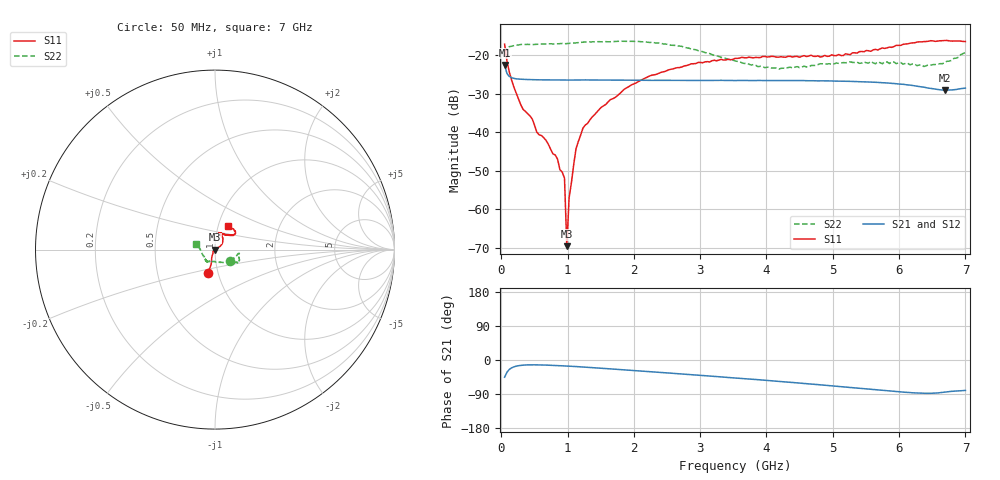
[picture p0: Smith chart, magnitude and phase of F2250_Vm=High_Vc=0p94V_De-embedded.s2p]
! Integrated Device Technology
! Corporate Headquarters
! 6024 Silver Creek Valley Road
! San Jose, CA 95138  USA
! Phone:  1-408-284-8200
! Toll Free:  1-800-223-1366
! Webpage:  http://www.idt.com/
! Timing and RF Division
! 515 Groton Road, Suite 102
! Westford, MA 01886-6024
! Device:  F2250
! Description: Voltage Variable RF Attenuator
! Frequency:  50.0 -  6000.00 MHz
! Package:  3x3 mm Thin QFN Plastic Package: 16 pin
! Ports:  2 RF, 3 DC
!  Pin  1  = GND
!  Pin  2  = NC
!  Pin  3  = RF1  = Port 1
!  Pin  4  = NC
!  Pin  5  = GND
!  Pin  6  = GND
!  Pin  7  = GND
!  Pin  8  = GND
!  Pin  9  = NC
!  Pin 10  = RF2  = Port 2
!  Pin 11  = NC
!  Pin 12  = GND
!  Pin 13  = GND
!  Pin 14  = VCNTRL
!  Pin 15  = VDD
!  Pin 16  = VMODE
! Vcntrl:  0.940 Volts
! Vmode:  +3.300 Volts
! Vdd:  +3.30  Volts
! Current:  1.318 mA
! Data:  The device was measured on a the F2250 evaluation board which has
!  individual transmission lines to the RF pins.  Data was collected
!  using a calibrated network analyzer.  The evaluation board was
!  de-embedded using a TRL calibration technique.
!  The reference plane is the edge of the package pin.
! Misc:  SN 10
!  Action Tracker AT0258
! Date Measured:  2014-11-26
! Date:  2015-10-15  MJV
! Note:
!  Integrated Device Technology supplies this data as a sample of measured
!  data at the package pin for this product.  Your particular data for this
!  product may vary.
!  Data was taken at 25 degrees C.
!  Integrated Device Technology reserves the right to change this data at anytime.
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# GHz S dB R 50
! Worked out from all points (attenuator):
!   201 points, 50 MHz to 7 GHz, reference 50 ohm
!   highest |S21| = -22.61 dB at 50 MHz (marker M1); lowest = -29.2 dB at 6.687 GHz (marker M2)
!   lowest |S11| = -69.6 dB at 988.2 MHz (marker M3), VSWR 1.00, Z = 50 - j0.0251 ohm
!   |S11| at or under -10 dB: start of sweep to end of sweep
!   |S22| runs from -23.7 to -16.4 dB; largest |S21 - S12| = 0.0002
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0.05  -17.20 -106.5  -22.61 -45.4  -22.62 -45.4  -19.62 -37.5
0.1195  -24.34 -108.4  -25.55 -25.2  -25.55 -25.1  -17.85 -12.2
0.29325  -32.89 -119.0  -26.29 -14.2  -26.29 -14.2  -17.29 -9.6
0.467  -36.62 -135.9  -26.42 -12.7  -26.42 -12.7  -17.32 -9.9
0.5365  -40.03 -141.6  -26.44 -12.8  -26.43 -12.8  -17.23 -11.2
0.6755  -42.17 -150.1  -26.46 -13.5  -26.46 -13.5  -17.14 -13.1
0.8145  -45.95 174.6  -26.47 -14.4  -26.49 -14.4  -17.15 -15.7
0.9535  -51.98 -174.4  -26.51 -15.6  -26.51 -15.6  -17.10 -18.0
0.98825  -69.59 -130.8  -26.50 -15.9  -26.52 -15.9  -17.05 -18.5
1.023  -57.03 24.2  -26.51 -16.3  -26.52 -16.3  -16.97 -18.7
1.12725  -44.29 23.8  -26.49 -17.3  -26.50 -17.3  -16.84 -20.2
1.2315  -38.99 23.1  -26.47 -18.5  -26.48 -18.5  -16.68 -22.0
1.5095  -33.56 31.1  -26.51 -21.8  -26.51 -21.9  -16.59 -24.3
1.857  -28.86 33.6  -26.54 -26.1  -26.55 -26.1  -16.44 -27.2
2.37825  -24.73 43.0  -26.57 -32.5  -26.59 -32.5  -16.89 -30.8
3.525  -20.89 70.0  -26.65 -47.4  -26.64 -47.4  -21.54 -58.1
4.18525  -20.56 76.3  -26.65 -56.3  -26.66 -56.3  -23.67 -93.0
4.7065  -20.35 71.1  -26.69 -64.0  -26.69 -64.0  -22.72 -114.4
5.85325  -17.96 39.6  -27.33 -81.7  -27.33 -81.8  -22.22 -128.3
6.3745  -16.53 40.3  -28.36 -87.9  -28.38 -87.9  -23.00 -146.3
6.68725  -16.25 47.2  -29.17 -85.0  -29.19 -85.0  -22.06 -177.1
7  -16.53 61.9  -28.60 -80.3  -28.59 -80.4  -19.39 164.5
